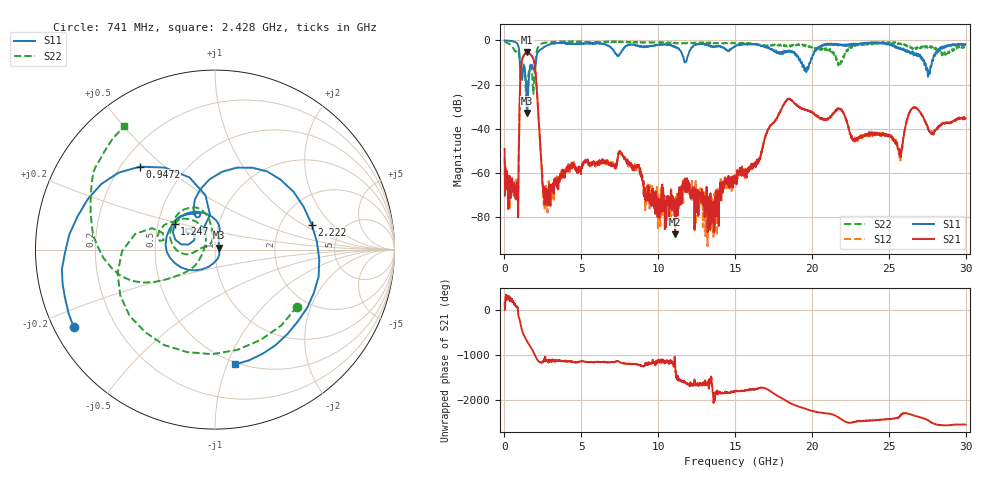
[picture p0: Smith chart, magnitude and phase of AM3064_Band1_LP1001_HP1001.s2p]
# Hz S DB R 50.0
!freq dBS11 angS11 dBS21 angS21 dBS12 angS12 dBS22 angS22
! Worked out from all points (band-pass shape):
!   1600 points, 10 MHz to 29.98 GHz, reference 50 ohm
!   highest |S21| = -5.40 dB at 1.472 GHz (marker M1); lowest = -87.7 dB at 11.11 GHz (marker M2)
!   |S21| within 3 dB of the highest: 1.161 GHz to 1.881 GHz (719.8 MHz wide, 47.3 % of centre)
!   lowest |S11| = -32.8 dB at 1.472 GHz (marker M3), VSWR 1.05, Z = 52 + j1.11 ohm
!   |S11| at or under -10 dB: 1.002 GHz to 2.041 GHz (1.039 GHz wide, 68.3 % of centre); 19.35 GHz to 19.89 GHz (545.4 MHz wide, 2.78 % of centre); 27.3 GHz to 27.8 GHz (495.7 MHz wide, 1.8 % of centre)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
!   |S22| runs from -27.6 to -0.3 dB; largest |S21 - S12| = 0.0073
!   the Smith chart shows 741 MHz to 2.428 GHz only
!   S11 on the Smith chart (normalised r, x): 741 MHz: 0.06, -0.26; 947.2 MHz: 0.28, +0.42; 1.247 GHz: 0.61, +0.19; 2.222 GHz: 2.98, +1.20; 2.428 GHz: 0.48, -1.07
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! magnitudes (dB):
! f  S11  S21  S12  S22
! 10 MHz  0.0  -49.1  -53.5  -0.3
! 741 MHz  -0.9  -68.0  -69.2  -5.1
! 947.2 MHz  -4.1  -43.7  -43.4  -5.7
! 1.247 GHz  -11.5  -7.0  -6.9  -11.0
! 1.472 GHz  -32.8  -5.4  -5.4  -22.5
! 1.922 GHz  -13.3  -9.4  -9.3  -19.0
! 2.222 GHz  -5.1  -35.2  -35.0  -2.6
! 2.428 GHz  -3.8  -58.9  -58.3  -1.4
! 2.747 GHz  -2.4  -70.0  -70.3  -0.9
! 5.015 GHz  -1.4  -57.6  -57.7  -0.6
! 7.564 GHz  -5.7  -51.0  -51.0  -0.5
! 10 GHz  -2.0  -71.6  -69.3  -1.0
! 11.11 GHz  -2.9  -87.7  -74.6  -1.3
! 13.67 GHz  -2.8  -79.1  -69.1  -1.2
! 15 GHz  -2.7  -62.8  -62.3  -1.4
! 18.38 GHz  -4.9  -26.8  -26.8  -2.7
! 19.99 GHz  -8.3  -32.5  -32.6  -3.0
! 25 GHz  -1.5  -43.5  -43.0  -1.0
! 25.76 GHz  -3.9  -52.9  -54.4  -1.3
! 26.63 GHz  -6.8  -30.3  -30.3  -3.1
! 27.56 GHz  -16.3  -40.3  -39.5  -2.7
! 29.98 GHz  -1.7  -35.5  -35.6  -3.1
